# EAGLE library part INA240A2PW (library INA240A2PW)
80V, Low-/High-Side, Bi-Directional, Zero-Drift, Current Sense Amp w/Enhanced PWM Rejection Source: Datasheet
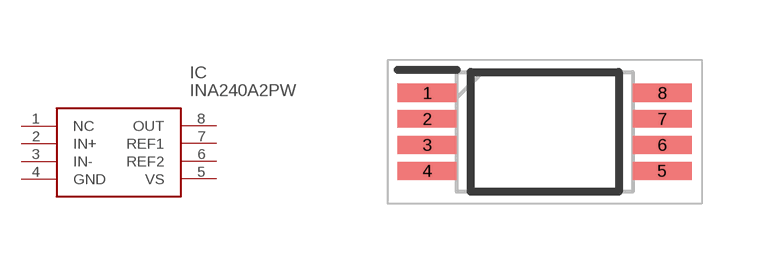
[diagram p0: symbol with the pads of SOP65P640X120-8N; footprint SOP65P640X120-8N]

Designator prefix IC

## INA240A2PW (Arrow_Part_Number: INA240A2PW; Arrow_Price-Stock: https://www.arrow.com/en/products/ina240a2pw/texas-instruments?region=nac; Description: 80V, Low-/High-Side, Bi-Directional, Zero-Drift, Current Sense Amp w/Enhanced PWM Rejection; Height: 1.2mm; Manufacturer_Name: Texas Instruments; Manufacturer_Part_Number: INA240A2PW; Mouser_Part_Number: 595-INA240A2PW; Mouser_Price-Stock: https://www.mouser.co.uk/ProductDetail/Texas-Instruments/INA240A2PW?qs=aVyJF2WnouTiD4LDXEZ4Dw%3D%3D)  [SOP65P640X120-8N]
1  NC  nc
2  IN+
3  IN-
4  GND
5  VS
6  REF2
7  REF1
8  OUT

## Footprint SOP65P640X120-8N (pad centres in mm)
PW0008A
smd 1.475 x 0.45: 1 -2.938,0.975; 2 -2.938,0.325; 3 -2.938,-0.325; 4 -2.938,-0.975; 5 2.938,-0.975; 6 2.938,-0.325; 7 2.938,0.325; 8 2.938,0.975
